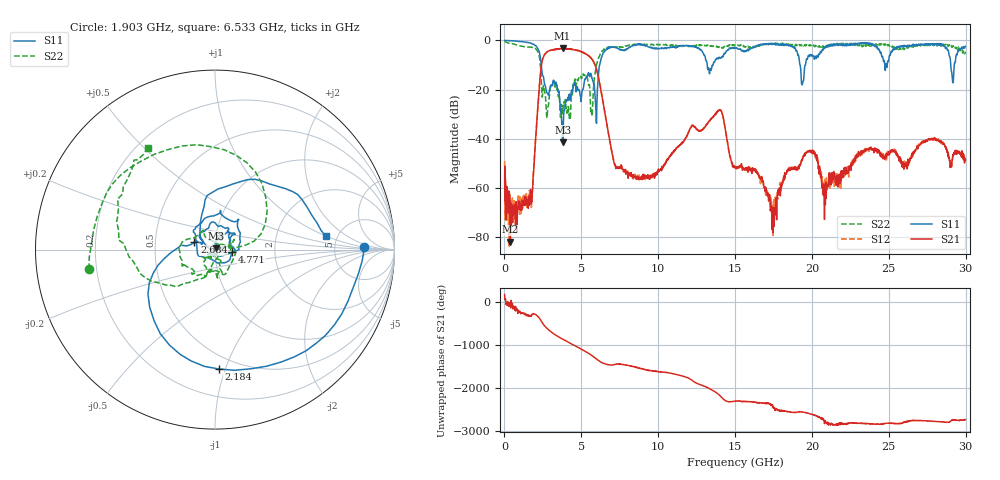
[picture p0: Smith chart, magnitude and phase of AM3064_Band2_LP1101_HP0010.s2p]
# Hz S DB R 50.0
!freq dBS11 angS11 dBS21 angS21 dBS12 angS12 dBS22 angS22
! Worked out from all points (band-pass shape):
!   1600 points, 10 MHz to 29.98 GHz, reference 50 ohm
!   highest |S21| = -3.29 dB at 3.777 GHz (marker M1); lowest = -81.9 dB at 384.9 MHz (marker M2)
!   |S21| within 3 dB of the highest: 2.567 GHz to 5.466 GHz (2.899 GHz wide, 72.2 % of centre)
!   lowest |S11| = -41.5 dB at 3.796 GHz (marker M3), VSWR 1.02, Z = 50.4 + j0.763 ohm
!   |S11| at or under -10 dB: 2.396 GHz to 6.193 GHz (3.798 GHz wide, 88.4 % of centre); 13.19 GHz to 13.57 GHz (380.2 MHz wide, 2.84 % of centre); 19.23 GHz to 19.58 GHz (351.6 MHz wide, 1.81 % of centre)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
!   |S22| runs from -32.2 to -0.2 dB; largest |S21 - S12| = 0.018
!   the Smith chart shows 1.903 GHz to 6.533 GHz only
!   S11 on the Smith chart (normalised r, x): 1.903 GHz: 11, +1; 2.184 GHz: 0.40, -0.95; 2.634 GHz: 0.79, +0.07; 4.771 GHz: 1.21, -0.03; 6.533 GHz: 4.03, +0.99
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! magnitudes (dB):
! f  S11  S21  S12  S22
! 10 MHz  0.0  -55.0  -49.1  -0.2
! 384.9 MHz  -0.2  -81.9  -75.1  -1.3
! 1.641 GHz  -1.0  -64.5  -61.5  -2.8
! 1.903 GHz  -1.6  -52.9  -51.9  -3.0
! 2.184 GHz  -3.5  -25.9  -26.0  -4.8
! 2.634 GHz  -18.2  -5.6  -5.6  -21.4
! 3.777 GHz  -40.3  -3.3  -3.3  -29.8
! 3.796 GHz  -41.5  -3.4  -3.3  -28.6
! 4.771 GHz  -20.2  -4.2  -4.1  -16.4
! 5.015 GHz  -22.6  -4.7  -4.7  -15.6
! 5.671 GHz  -15.0  -7.5  -7.5  -29.5
! 5.952 GHz  -28.8  -11.1  -11.1  -10.9
! 6.533 GHz  -4.1  -29.4  -29.4  -3.3
! 7.283 GHz  -3.1  -51.9  -51.9  -2.6
! 10 GHz  -3.4  -52.7  -53.1  -1.8
! 13.97 GHz  -6.9  -28.5  -28.3  -2.8
! 15 GHz  -3.0  -51.7  -51.9  -1.9
! 17.46 GHz  -1.2  -68.8  -67.4  -1.4
! 19.99 GHz  -5.8  -45.3  -45.4  -1.8
! 20.89 GHz  -2.4  -58.2  -58.7  -2.8
! 25 GHz  -8.0  -45.5  -45.6  -1.8
! 29.98 GHz  -2.4  -48.8  -48.8  -4.6
